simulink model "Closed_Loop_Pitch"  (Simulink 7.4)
settings: Solver=ode45  StartTime=0.0  StopTime=10.0  RelTol=1e-3
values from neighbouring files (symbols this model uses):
  Ap = Au([3,4,7,9,10],[3,4,7,9,10])    [Split.m]
  Bp = Bu([3,4,7,9,10],                      [4,8, 10,12,13,15,16,17,18,23,25,27,31,32,33,34])    [Split.m]
  Cp = Cu([3,4,7,9,10,12,14, 16,18,19,21,22,23,24,29,31,33,37,38,39,40],         [3,4,7,9,10])    [Split.m]
  Dp = Du([3,4,7,9,10,12,14, 16,18,19,21,22,23,24,29,31,33,37,38,39,40],                      [4,8, 10,12,13,15,16,17,18,23,25,27,31,32,33,34])    [Split.m]
  npu = 14    [run.m]
undefined symbols (not defined in the file or in its folder): Kp

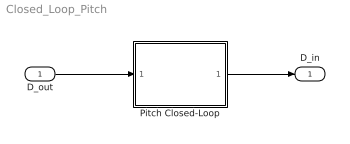
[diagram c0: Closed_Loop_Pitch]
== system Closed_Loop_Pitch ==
  D_out : Inport  OutDataType=sfix(16)  OutScaling=2^0
  Pitch Closed-Loop : Subsystem
  D_in : Outport  OutDataType=sfix(16)  OutScaling=2^0
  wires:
  Pitch Closed-Loop/1(D_in) -> D_in/1
  D_out/1 -> Pitch Closed-Loop/1(D_out)

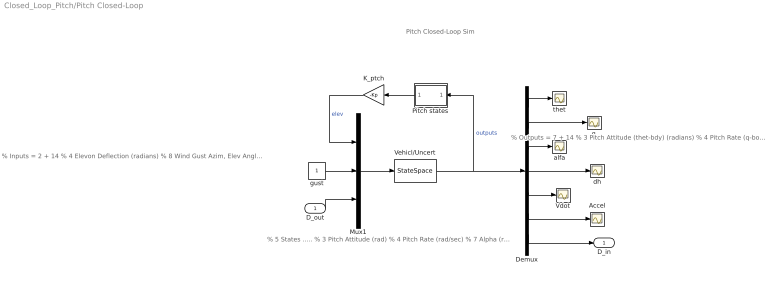
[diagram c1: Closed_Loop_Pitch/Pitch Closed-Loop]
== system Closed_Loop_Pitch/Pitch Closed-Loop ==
  note: Pitch Closed-Loop Sim
  note: % 5 States ..... % 3 Pitch Attitude (rad) % 4 Pitch Rate (rad/sec) % 7 Alpha (rad) % 9 Delta_Altitude (ft) % 10 Delta_veloc (ft/sec)
  note: % Inputs = 2 + 14 % 4 Elevon Deflection (radians) % 8 Wind Gust Azim, Elev Angles=(-135, 90) (deg) % Pitch Variations= 14 % 10 Cm_alfa : -166.667 % Variation % 12 Ca_alpha : -22.222 % Variation % 13 Cz_alpha : -10.000 % Variation % 15 Cm_0 : -50.000 % Variation % 16 CZ_0 : -2.857 % Variation % 17 Cm_q : -40.000 % Variation % 18 Cz_q : -20.000 % Variation % 23 CA_0 : -952.381 % Variation % 25 I_yy : 3.333 % Variation % 27 Xcg locat: -1.766 % Variation % 31 Zcg locat: 0.5000 Addit. Variat. % 32 Ca_surf 1: -18.182 % Variation % 33 Cz_surf 1: -16.667 % Variation % 34 Cm_surf 1: 13.333 % Variation
  note: % Outputs = 7 + 14 % 3 Pitch Attitude (thet-bdy) (radians) % 4 Pitch Rate (q-body) (rad/sec) % 7 Angle of attack, alfa, (radians) % 9 Change in Altitude, delta-h, (feet) % 10 Forward Acceleration (V-dot) (ft/sec) % 12 CG Acceleration along X axis, (ft/sec^2) % 14 CG Acceleration along Z axis, (ft/sec^2) % Pitch Variations= 14 % 16 Cm_alfa : -166.667 % Variation % 18 Ca_alpha : -22.222 % Variation % 19 Cz_alpha : -10.000 % Variation % 21 Cm_0 : -50.000 % Variation % 22 CZ_0 : -2.857 % Variation % 23 Cm_q : -40.000 % Variation % 24 Cz_q : -20.000 % Variation % 29 CA_0 : -952.381 % Variation % 31 I_yy : 3.333 % Variation % 33 Xcg locat: -1.766 % Variation % 37 Zcg locat: 0.5000 Addit. Variat. % 38 Ca_surf 1: -18.182 % Variation % 39 Cz_surf 1: -16.667 % Variation % 40 Cm_surf 1: 13.333 % Variation
  D_out : Inport  OutDataType=fixdt(1, 16)  OutScaling=2^0
  Accel : Scope
  Demux : Demux  Outputs="[1,1,1,1,1,  2,  npu]"
  K_ptch : Gain  Gain=-Kp  Multiplication=Matrix(K*u)  ParameterDataType=sfix(16)  ParameterScaling=2^0  OutDataType=sfix(16)  OutScaling=2^0
  Mux1 : Mux  Inputs=[1,1, npu]
  Pitch states : Subsystem
  Vdot : Scope
  Vehicl/Uncert : StateSpace  A=Ap  B=Bp  C=Cp  D=Dp
  alfa : Scope
  dh : Scope
  gust : Constant  OutDataType=sfix(16)  OutScaling=2^0
  q : Scope
  thet : Scope
  D_in : Outport  OutDataType=sfix(16)  OutScaling=2^0
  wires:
  Vehicl/Uncert/1 -> Demux/1, Pitch states/1(stat)  "outputs"
  Demux/1 -> thet/1
  Demux/2 -> q/1
  Demux/3 -> alfa/1
  Demux/4 -> dh/1
  Demux/5 -> Vdot/1
  Mux1/1 -> Vehicl/Uncert/1
  Demux/6 -> Accel/1
  Demux/7 -> D_in/1
  Pitch states/1(xp) -> K_ptch/1
  K_ptch/1 -> Mux1/1  "elev"
  gust/1 -> Mux1/2
  D_out/1 -> Mux1/3

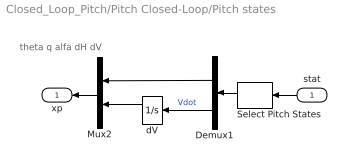
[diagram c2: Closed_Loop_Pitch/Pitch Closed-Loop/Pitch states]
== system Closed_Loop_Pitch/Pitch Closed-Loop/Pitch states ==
  note: theta q alfa dH dV
  stat : Inport  OutDataType=sfix(16)  OutScaling=2^0
  Demux1 : Demux  Outputs=[4,1]
  Mux2 : Mux  Inputs=[4, 1]
  Select Pitch States : Selector  InputPortWidth=7+npu  IndexOptions=Index vector (dialog)  Indices=[1,2,3,4,5]  OutputSizes=1
  dV : Integrator
  xp : Outport  OutDataType=sfix(16)  OutScaling=2^0
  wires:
  Select Pitch States/1 -> Demux1/1
  Demux1/2 -> dV/1  "Vdot"
  Demux1/1 -> Mux2/1
  Mux2/1 -> xp/1
  stat/1 -> Select Pitch States/1
  dV/1 -> Mux2/2
